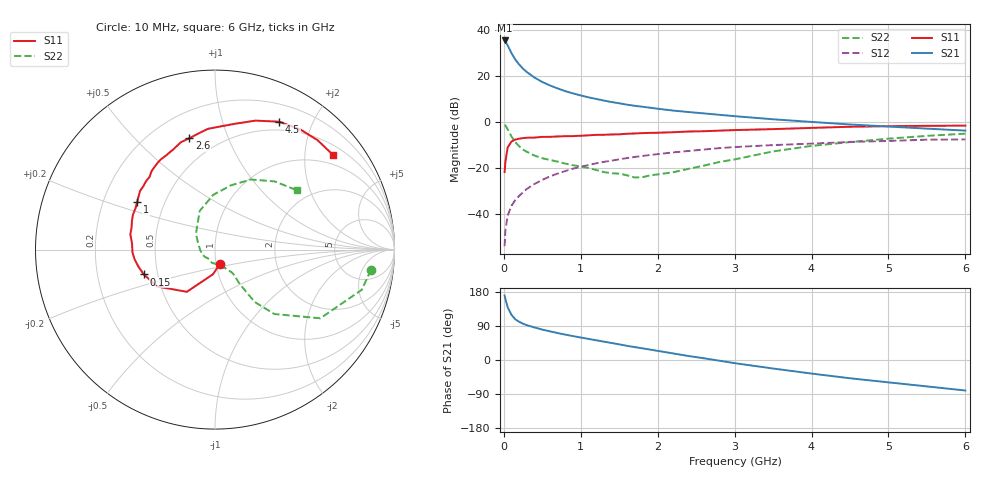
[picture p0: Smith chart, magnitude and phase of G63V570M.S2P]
! SIEMENS Small Signal Semiconductors
! BFG193
! Si NPN RF Bipolar Junction Transistor in SOT223
! VCE = 3.5 V  IC = 70 mA
! Common Emitter S-Parameters:  August  1996
# GHz  S  MA  R  50
!  f  S11  S21  S12  S22
! GHz  MAG  ANG  MAG  ANG  MAG  ANG  MAG  ANG
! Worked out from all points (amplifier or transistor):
!   36 points, 10 MHz to 6 GHz, reference 50 ohm
!   highest |S21| = 35.6 dB at 10 MHz (marker M1)
!   |S21| within 3 dB of that: start of sweep to 62.27 MHz
!   unconditionally stable (mu >= 1): 324.2 MHz to 2.362 GHz
!   at 250 MHz: K = 0.97, MSG = 26.9 dB, |S12| = -30.4 dB
!   at 1.4 GHz: K = 1.05, MAG = 11.4 dB, |S12| = -16.7 dB
!   at 6 GHz: K = 0.91, MSG = 1.9 dB, |S12| = -7.5 dB
!   S11 on the Smith chart (normalised r, x): 10 MHz: 1.04, -0.16; 150 MHz: 0.42, -0.14; 1 GHz: 0.35, +0.25; 2.6 GHz: 0.35, +0.73; 4.5 GHz: 0.40, +1.55; 6 GHz: 0.74, +2.68
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0.01  0.0825 -70.1  60.39 170.1  0.002 84.7  0.8759 -7.4
0.02  0.1374 -94.5  57.75 161.3  0.0044 76.7  0.8482 -15.3
0.05  0.2827 -123.7  47.03 139.0  0.0093 72.4  0.7007 -33.1
0.1  0.3815 -147.4  31.89 119.0  0.0152 67.9  0.4885 -47.3
0.15  0.4202 -160.8  23.07 107.2  0.0204 68.5  0.3671 -52.8
0.2  0.4374 -167.6  18.01 100.7  0.025 70.1  0.301 -53.5
0.25  0.4509 -173.0  14.62 95.7  0.0301 70.6  0.253 -54.0
0.3  0.4599 -177.8  12.34 91.8  0.0354 71.4  0.2266 -54.2
0.4  0.4638 175.6  9.362 85.8  0.0454 70.7  0.1872 -53.5
0.5  0.4793 169.8  7.527 80.2  0.0557 70.1  0.1644 -53.1
0.6  0.4808 165.2  6.32 75.6  0.0662 69.0  0.151 -54.5
0.7  0.4902 160.7  5.439 71.1  0.0764 67.7  0.1385 -57.1
0.8  0.4971 156.8  4.749 67.0  0.0867 65.4  0.1256 -59.5
1  0.5086 148.4  3.827 59.3  0.1071 61.8  0.1089 -66.0
1.1  0.5184 145.3  3.485 55.7  0.1169 59.9  0.1009 -72.5
1.6  0.5614 129.1  2.416 37.4  0.1657 48.7  0.0701 -110.5
2.2  0.6059 112.3  1.797 17.4  0.2205 35.0  0.0813 -175.5
2.6  0.6368 102.9  1.558 4.6  0.2543 26.1  0.1135 150.4
3.5  0.7081 81.4  1.16 -22.5  0.3181 3.3  0.2316 111.6
4.5  0.797 63.4  0.893 -48.2  0.3726 -17.0  0.3696 75.9
5.5  0.8356 46.8  0.726 -69.7  0.417 -40.5  0.505 48.8
6  0.8434 38.5  0.657 -80.5  0.422 -54.0  0.5641 35.8
